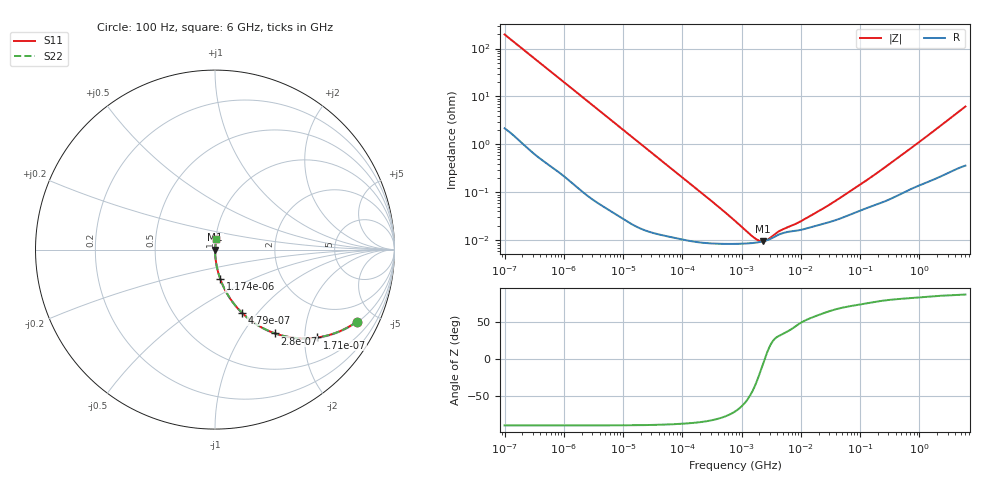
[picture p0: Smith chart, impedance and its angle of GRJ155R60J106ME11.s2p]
!Murata Part Number: GRJ155R60J106ME11
!These Parameters are Measured in Series Mode Connection
!Data Generated on Jun 19, 2026
!  o--ll--o
!Port1  Port2
!  o------o
!Operation Temp=25[degC], DC Bias Voltage=0[V]
!Freq. Start=100[Hz] Stop=6[GHz] 401[Steps]
# Hz S RI R 50
!Freq.(Hz) S11(Real) S11(Imag) S21(Real) S21(Imag) S12(Real) S12(Imag) S22(Real) S22(Imag)
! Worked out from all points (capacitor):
!   401 points, 100 Hz to 6 GHz, reference 50 ohm
!   read as one part in series: C = 8.08 uF near 109 Hz
!   lowest |Z| = 9.57 mohm at 2.269 MHz (marker M1)
!   series resonance near 2.456 MHz, so ESL is about 520 pH
!   S11 on the Smith chart (normalised r, x): 100 Hz: 1.04, -3.93; 171 Hz: 1.02, -2.31; 280 Hz: 1.01, -1.41; 479 Hz: 1.01, -0.83; 1.174 kHz: 1.00, -0.34; 6 GHz: 1.01, +0.12
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100  0.7916 -0.4007  0.2084 0.4007  0.2084 0.4007  0.7916 -0.4007
120  0.7279 -0.4395  0.2721 0.4395  0.2721 0.4395  0.7279 -0.4395
171  0.5701 -0.4897  0.4299 0.4897  0.4299 0.4897  0.5701 -0.4897
280  0.3349 -0.4669  0.6651 0.4669  0.6651 0.4669  0.3349 -0.4669
479  0.1491 -0.3511  0.8509 0.3511  0.8509 0.3511  0.1491 -0.3511
717  0.074 -0.2564  0.926 0.2564  0.926 0.2564  0.074 -0.2564
1174  0.0299 -0.1649  0.9701 0.1649  0.9701 0.1649  0.0299 -0.1649
2008  0.0109 -0.0987  0.9891 0.0987  0.9891 0.0987  0.0109 -0.0987
6433  0.00138 -0.0313  0.9986 0.0313  0.9986 0.0313  0.00138 -0.0313
40335  0.000158 -0.00506  0.9998 0.00506  0.9998 0.00506  0.000158 -0.00506
774597  8.44e-05 -0.000241  0.9999 0.000241  0.9999 0.000241  8.44e-05 -0.000241
1658239  8.88e-05 -6.75e-05  0.9999 6.75e-05  0.9999 6.75e-05  8.88e-05 -6.75e-05
1896632  9.09e-05 -4.37e-05  0.9999 4.37e-05  0.9999 4.37e-05  9.09e-05 -4.37e-05
2268635  9.48e-05 -1.31e-05  0.9999 1.31e-05  0.9999 1.31e-05  9.48e-05 -1.31e-05
2837864  0.000103 2.37e-05  0.9999 -2.37e-05  0.9999 -2.37e-05  0.000103 2.37e-05
4440638  0.000135 8.32e-05  0.9999 -8.32e-05  0.9999 -8.32e-05  0.000135 8.32e-05
8692127  0.00016 0.000163  0.9998 -0.000163  0.9998 -0.000163  0.00016 0.000163
1.555665e7  0.000191 0.000281  0.9998 -0.000281  0.9998 -0.000281  0.000191 0.000281
4.983056e7  0.000296 0.000764  0.9997 -0.000764  0.9997 -0.000764  0.000296 0.000764
3.124326e8  0.000727 0.00383  0.9993 -0.00383  0.9993 -0.00383  0.000727 0.00383
1.873145e9  0.00232 0.0201  0.9977 -0.0201  0.9977 -0.0201  0.00232 0.0201
6e9  0.00735 0.061  0.9927 -0.061  0.9927 -0.061  0.00735 0.061
